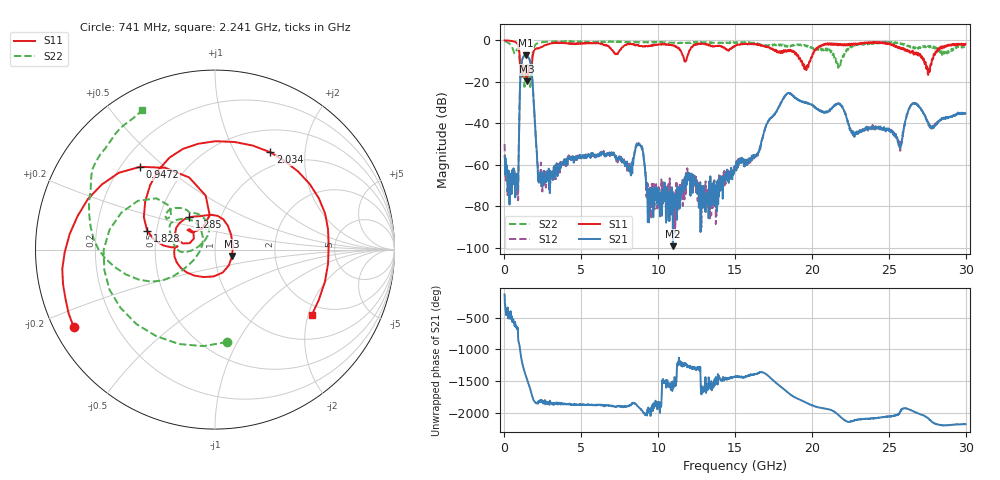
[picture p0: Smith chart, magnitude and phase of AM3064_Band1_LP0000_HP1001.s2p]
# Hz S DB R 50.0
!freq dBS11 angS11 dBS21 angS21 dBS12 angS12 dBS22 angS22
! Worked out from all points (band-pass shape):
!   1600 points, 10 MHz to 29.98 GHz, reference 50 ohm
!   highest |S21| = -7.17 dB at 1.378 GHz (marker M1); lowest = -99.2 dB at 10.96 GHz (marker M2)
!   |S21| within 3 dB of the highest: 1.13 GHz to 1.672 GHz (542.9 MHz wide, 38.7 % of centre)
!   lowest |S11| = -19.8 dB at 1.472 GHz (marker M3), VSWR 1.23, Z = 60.4 - j4.35 ohm
!   |S11| at or under -10 dB: 1.002 GHz to 1.801 GHz (799.8 MHz wide, 57.1 % of centre); 19.34 GHz to 19.89 GHz (546.6 MHz wide, 2.79 % of centre); 27.3 GHz to 27.79 GHz (496.1 MHz wide, 1.8 % of centre)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
!   |S22| runs from -22.5 to -0.2 dB; largest |S21 - S12| = 0.0047
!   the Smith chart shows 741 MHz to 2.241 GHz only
!   S11 on the Smith chart (normalised r, x): 741 MHz: 0.06, -0.26; 947.2 MHz: 0.28, +0.42; 1.285 GHz: 0.71, +0.27; 1.828 GHz: 0.44, +0.11; 2.034 GHz: 0.79, +1.40; 2.241 GHz: 1.67, -2.11
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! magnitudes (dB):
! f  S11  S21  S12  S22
! 10 MHz  -0.1  -56.0  -50.0  -0.2
! 741 MHz  -0.9  -67.8  -64.1  -5.7
! 947.2 MHz  -4.1  -44.0  -44.2  -5.9
! 1.116 GHz  -16.2  -10.7  -10.6  -11.4
! 1.285 GHz  -12.8  -7.4  -7.4  -21.0
! 1.378 GHz  -14.5  -7.2  -7.2  -14.2
! 1.472 GHz  -19.8  -7.5  -7.4  -11.2
! 1.828 GHz  -8.1  -20.4  -20.3  -6.8
! 2.034 GHz  -4.1  -46.0  -46.6  -1.9
! 2.241 GHz  -3.7  -68.6  -68.0  -1.1
! 5.015 GHz  -1.4  -56.1  -56.6  -0.8
! 8.763 GHz  -2.7  -50.0  -49.9  -1.1
! 9.382 GHz  -2.8  -79.5  -76.7  -0.8
! 10 GHz  -2.0  -75.0  -77.4  -0.9
! 10.96 GHz  -2.3  -99.2  -78.8  -1.1
! 15 GHz  -2.8  -60.6  -62.1  -1.3
! 18.36 GHz  -5.4  -25.8  -25.7  -2.9
! 19.99 GHz  -8.1  -31.1  -31.2  -3.5
! 25 GHz  -1.3  -43.5  -43.0  -1.0
! 26.63 GHz  -6.9  -30.4  -30.2  -3.2
! 27.56 GHz  -16.6  -39.6  -40.3  -2.7
! 29.98 GHz  -1.7  -35.3  -35.4  -3.1
